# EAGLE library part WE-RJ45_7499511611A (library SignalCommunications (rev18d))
Order Code 7499511611A Design THT xBase-T 10/100/1000 Base-T Ports 1x1 Application PoE+ HPLE Tab Position Up LED (Left-Right) GREEN/ORANGE-YELLOW EMI Fingers YES Details see: http://katalog.we-online.de/en/pbs/WE-LAN_RJ45/7499511611A? Updated by Yingchun Shan 2016-08-30 2016(C) Würth Elektronik
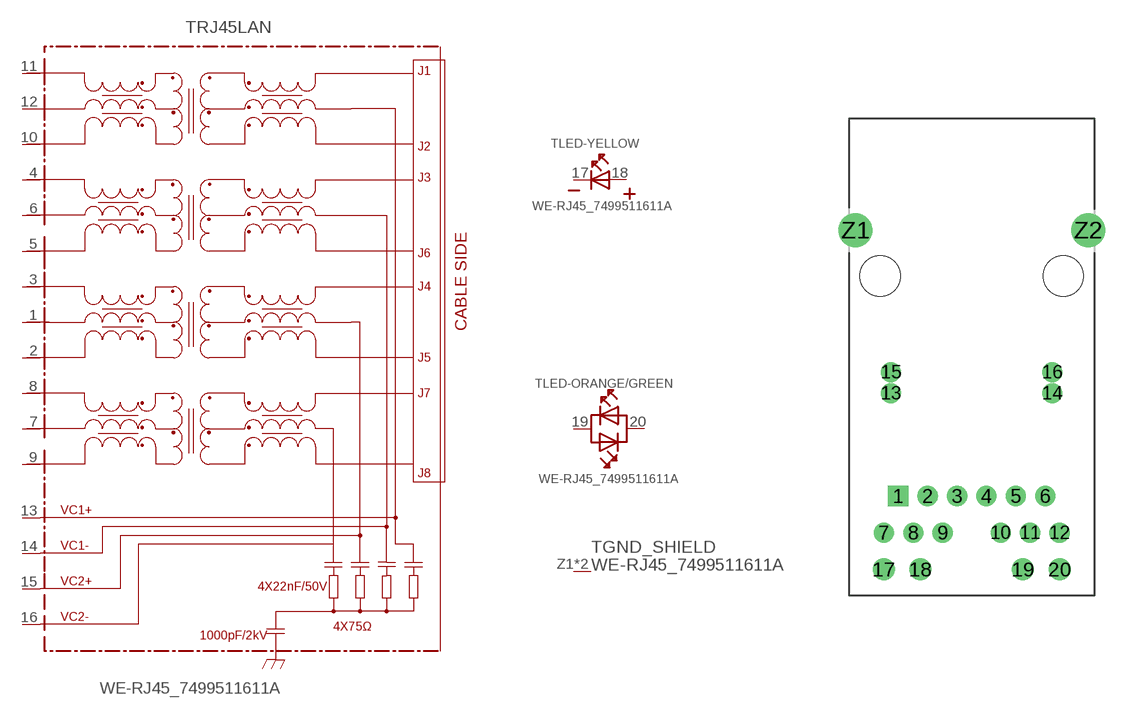
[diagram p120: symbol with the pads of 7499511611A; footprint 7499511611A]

Designator prefix T; gates RJ45LAN=7499511611A LED-YELLOW=LED-2PIN LED-ORANGE/GREEN=LED-DUAL GND_SHIELD=GND_PIN

## WE-RJ45_7499511611A (COMPANY-URL: http://www.we-online.de; CREATED-BY: Christin Zierenner; CREATED-DATE: AUG 2012; DATASHEET-URL: http://katalog.we-online.de/kataloge/eisos/media/pdf/7499511611A.pdf; MANUFACTURER: Würth Elektronik eiSos GmbH)  [7499511611A]
1  RJ45LAN:1
2  RJ45LAN:2
3  RJ45LAN:3
4  RJ45LAN:4
5  RJ45LAN:5
6  RJ45LAN:6
7  RJ45LAN:7
8  RJ45LAN:8
9  RJ45LAN:9
10  RJ45LAN:10
11  RJ45LAN:11
12  RJ45LAN:12
13  RJ45LAN:VC1+  pwr
14  RJ45LAN:VC1-  pwr
15  RJ45LAN:VC2+  pwr
16  RJ45LAN:VC2-  pwr
17  LED-YELLOW:K  pas
18  LED-YELLOW:A  pas
19  LED-ORANGE/GREEN:AK1  pas
20  LED-ORANGE/GREEN:AK2  pas
Z1  GND_SHIELD:1  pwr
Z2  GND_SHIELD:1  pwr

## Footprint 7499511611A (pad centres in mm)
MAX HEIGHT=13.87mm PORTS----1X1 LED --YES
drill 0.89 square: 1 -5.095,-15.24
drill 0.89: 2 -3.055,-15.24; 3 -1.015,-15.24; 4 1.015,-15.24; 5 3.055,-15.24; 6 5.095,-15.24; 7 -6.09,-17.78; 8 -4.05,-17.78; 9 -2.01,-17.78; 10 2.01,-17.78; 11 4.05,-17.78; 12 6.09,-17.78
drill 0.89 pad 1.27: 13 -5.59,-8.12; 14 5.59,-8.12; 15 -5.59,-6.66; 16 5.59,-6.66
drill 1.02: 17 -6.095,-20.32; 18 -3.555,-20.32; 19 3.555,-20.32; 20 6.095,-20.32
drill 1.57: Z1 -8.065,3.18; Z2 8.065,3.18
hole 2.8 at -6.35,0
hole 2.8 at 6.35,0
